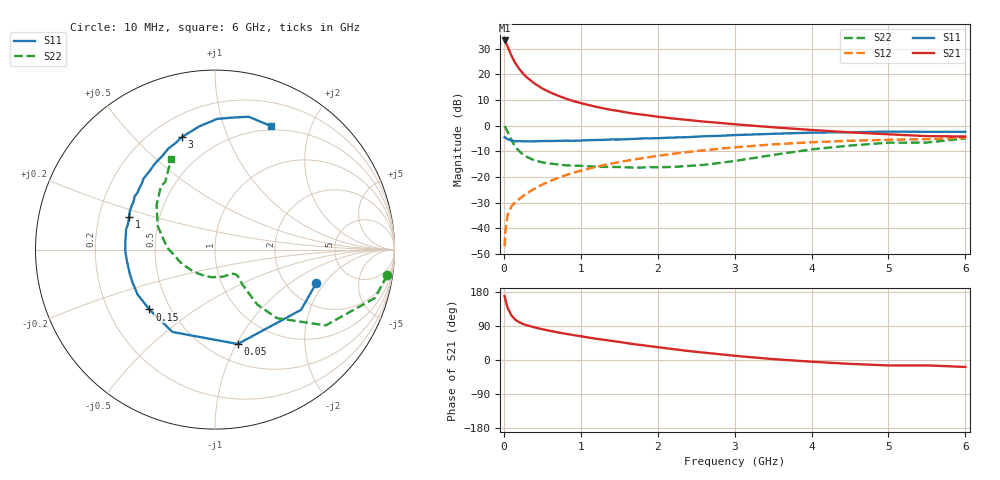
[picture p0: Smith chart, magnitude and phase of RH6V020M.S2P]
! SIEMENS Small Signal Semiconductors
! BFR106
! Si NPN RF Bipolar Junction Transistor in SOT23
! VCE = 6 V  IC = 20 mA
! Common Emitter S-Parameters:  August  1996
# GHz  S  MA  R  50
!  f  S11  S21  S12  S22
! GHz  MAG  ANG  MAG  ANG  MAG  ANG  MAG  ANG
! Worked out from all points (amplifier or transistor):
!   36 points, 10 MHz to 6 GHz, reference 50 ohm
!   highest |S21| = 33.1 dB at 10 MHz (marker M1)
!   |S21| within 3 dB of that: start of sweep to 57.24 MHz
!   unconditionally stable (mu >= 1): 374.9 MHz to 2.099 GHz
!   at 250 MHz: K = 0.88, MSG = 23.8 dB, |S12| = -27.4 dB
!   at 1.4 GHz: K = 1.06, MAG = 8.9 dB, |S12| = -14.8 dB
!   at 6 GHz: K = 0.99, MSG = 0.2 dB, |S12| = -4.7 dB
!   S11 on the Smith chart (normalised r, x): 10 MHz: 2.89, -1.66; 50 MHz: 0.68, -1.01; 150 MHz: 0.38, -0.34; 1 GHz: 0.33, +0.16; 3 GHz: 0.32, +0.70; 6 GHz: 0.46, +1.46
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0.01  0.5948 -18.2  45.38 168.8  0.0045 84.3  0.9693 -8.5
0.02  0.5853 -35.0  43.22 159.6  0.0089 75.7  0.9314 -16.8
0.05  0.5411 -76.4  34.06 137.1  0.0185 61.9  0.7478 -34.4
0.1  0.5165 -117.3  22.75 117.1  0.0271 54.7  0.5148 -47.9
0.15  0.4948 -137.6  16.32 106.0  0.0324 53.6  0.3864 -52.4
0.2  0.4986 -149.9  12.7 99.8  0.0373 56.3  0.3182 -52.3
0.25  0.4945 -158.2  10.27 94.9  0.0426 58.7  0.2714 -52.0
0.3  0.4937 -164.2  8.651 91.6  0.048 60.6  0.245 -51.8
0.4  0.4952 -173.2  6.577 86.1  0.0593 63.3  0.2105 -50.0
0.5  0.5002 -179.2  5.281 81.2  0.071 65.1  0.1922 -49.2
0.6  0.5011 175.3  4.445 77.0  0.0834 66.3  0.1828 -49.7
0.7  0.5035 170.8  3.843 72.9  0.0952 66.8  0.1755 -51.5
0.8  0.508 167.1  3.376 69.4  0.1079 66.6  0.1689 -53.0
1  0.5113 159.4  2.739 62.7  0.1324 66.0  0.1644 -57.4
1.1  0.5208 155.9  2.514 59.3  0.1449 65.3  0.162 -61.2
1.6  0.5431 140.6  1.795 44.5  0.2075 60.8  0.1541 -80.8
2.2  0.5846 124.9  1.373 28.8  0.2826 53.6  0.1569 -112.1
3  0.6528 106.6  1.062 11.1  0.3771 42.2  0.2046 -159.4
3.5  0.6924 97.2  0.927 2.4  0.4307 34.7  0.2682 177.1
4.5  0.7436 81.8  0.738 -10.2  0.5058 18.8  0.4086 142.9
5.5  0.7562 69.6  0.624 -14.2  0.5436 8.0  0.4678 126.4
6  0.7556 65.4  0.613 -18.4  0.5795 0.4  0.562 115.7
